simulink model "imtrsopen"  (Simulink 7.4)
settings: Solver=ode15s  StartTime=0  StopTime=4  MaxStep=1e-3  RelTol=1e-3
InitFcn:
  | imopendat
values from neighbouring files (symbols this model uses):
  Hi = str2num(get(h,'string'))    [imic33.m]
  ic = [fs0 fr0]    [imdef0vec.m]    (also in imdef1vec.m; imdef2vec.m = F; imic2.m = [phids phiqs phidr phiqr n0]'; imic3.m = [phids phiqs phidr phiqr n0]')
  L = length(t)    [fourierdec.m]    (also in IMabc2.m = [Lss  Lsr; IMabcf0.m = [Lss  Lsr; IMabcf1.m = [Lss  Lsr; IMcur0.m = [Ls  0   Lm  0)
  Rr = input('Rotor resistance)[default = 2] =')    [Actac.m]    (also in im1phase.m = 0.3; im3d.m = eval(get(hRr,'String')); IMabc2.m = 0.02; imabcparam.m = 0.408)
  Rs = eval(get(hRs,'String'))    [im3d.m]    (also in IMabc2.m = 0.01; imabcparam.m = 0.531; IMabcrun0.m = 0.531; IMabcrun1.m = 0.531)
  t1 = 2.0    (= 2)    [IMabc2.m]
  Tl0 = Is*conj(Is)*Req    [imdef0vec.m]    (also in imdef1vec.m; imdef2vec.m = Lm*(I(2)*I(3)-I(1)*I(4)); imdefrotflux.m; imdefSIvec1.m = Te0/To)
  vs = 1.0    (= 1)    [imdef0vec.m]    (also in imdef1vec.m; imdef2vec.m; imdefrotflux.m; imdefSIvec1.m)
  wo = 2*pi*freq0    [calc0.m]    (also in IMabc2.m = 376.991118431; imabcparam.m = 376.991118431; IMabcrun0.m = 376.991118431; IMabcrun1.m = 376.991118431)
undefined symbols (not defined in the file or in its folder): t2

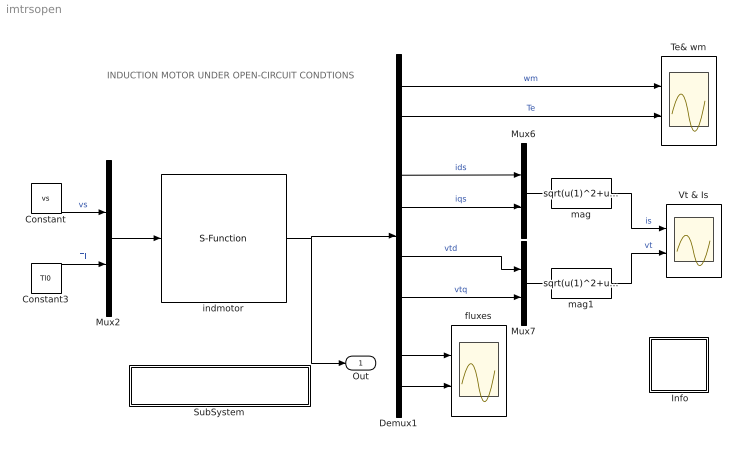
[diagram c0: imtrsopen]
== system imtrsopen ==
  note: INDUCTION MOTOR UNDER OPEN-CIRCUIT CONDTIONS
  " Info" : Subsystem
  Constant : Constant  Value=vs  OutDataType=sfix(16)  OutScaling=2^0
  Constant3 : Constant  Value=Tl0  OutDataType=sfix(16)  OutScaling=2^0
  Demux1 : Demux  Outputs=8
  Mux2 : Mux  Inputs=2
  Mux6 : Mux  Inputs=2
  Mux7 : Mux  Inputs=2
  SubSystem : Subsystem
  Te& wm : Scope  NumInputPorts=2
  Vt & Is : Scope  NumInputPorts=2
  fluxes : Scope  NumInputPorts=2
  indmotor : S-Function  FunctionName=imKmodopen  Parameters=Rs,Rr,L,Hi,wo,ic,t1,t2  EnableBusSupport=off
  mag : Fcn  Expr=sqrt(u(1)^2+u(2)^2)
  mag1 : Fcn  Expr=sqrt(u(1)^2+u(2)^2)
  Out : Outport
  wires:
  Mux6/1 -> mag/1
  Demux1/4 -> Mux6/2  "iqs"
  Demux1/3 -> Mux6/1  "ids"
  Demux1/5 -> Mux7/1  "vtd"
  Demux1/6 -> Mux7/2  "vtq"
  Mux7/1 -> mag1/1
  mag/1 -> Vt & Is/1  "is"
  Demux1/2 -> Te& wm/2  "Te"
  Mux2/1 -> indmotor/1
  indmotor/1 -> Demux1/1, Out/1
  mag1/1 -> Vt & Is/2  "vt"
  Demux1/1 -> Te& wm/1  "wm"
  Constant/1 -> Mux2/1  "vs"
  Constant3/1 -> Mux2/2  "Tl"
  Demux1/7 -> fluxes/1
  Demux1/8 -> fluxes/2

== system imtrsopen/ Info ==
  note: This demo simulates the running of an induction motor when the supply voltage is removed and then reapplied (Residual voltage)

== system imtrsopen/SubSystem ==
